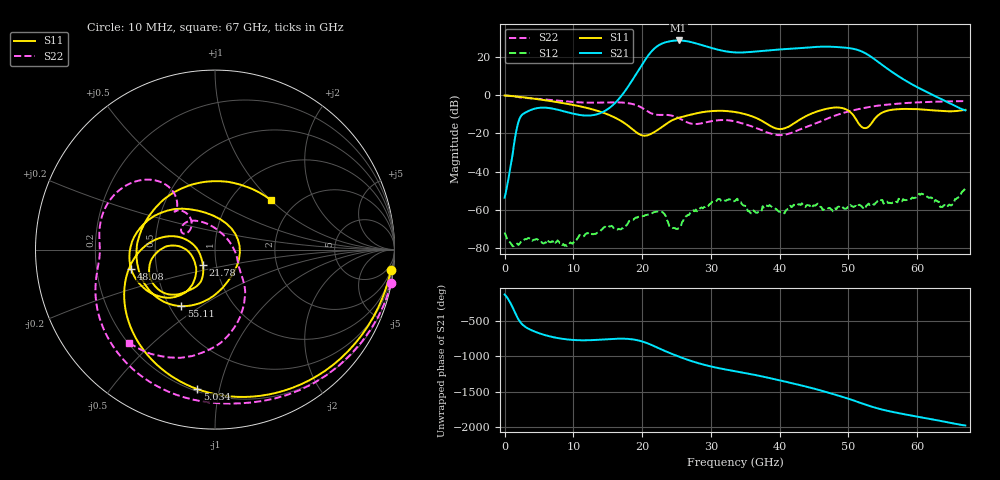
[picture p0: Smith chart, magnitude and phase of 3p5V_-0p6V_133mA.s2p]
! MARKI MICROWAVE INC.
! Date:  10/23/18
! Model Number:  AMM-6702CH
! Description:  2-port Small Signal S-parameter data for AMM-6702CH
! Frequency Range:  10 MHz to 67 GHz
! Port Configuration:  PORT 1: Input
!  PORT 2: Output
! Bias Condition: Vd = +3.5V, Vg = -0.6V
! AMM-6702CH s2p files are only valid for small signal conditions (below -5 dBm input power)
!S2P File: Measurements: Mag<S11> Ang<S11>, Mag<S21> Ang<S21>, Mag<S12> Ang<S12>, Mag<S22> Ang<S22>!row 1
# Hz S  dB  R 50
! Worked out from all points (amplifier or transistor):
!   401 points, 10 MHz to 67 GHz, reference 50 ohm
!   highest |S21| = 28.8 dB at 25.3 GHz (marker M1)
!   |S21| within 3 dB of that: 22.21 GHz to 29.21 GHz (7 GHz wide, 27.2 % of centre)
!   unconditionally stable (mu >= 1): start of sweep to end of sweep
!   at 11.06 GHz: K = 3267.83, MAG = -6.6 dB, |S12| = -73.4 dB
!   at 33.51 GHz: K = 18.14, MAG = 23.3 dB, |S12| = -55.3 dB
!   at 67 GHz: K = 135.82, MAG = -4.0 dB, |S12| = -48.5 dB
!   S11 on the Smith chart (normalised r, x): 10 MHz: 2, -17; 5.034 GHz: 0.21, -0.86; 21.78 GHz: 0.86, -0.15; 48.08 GHz: 0.36, -0.10; 55.11 GHz: 0.57, -0.42; 67 GHz: 1.51, +1.00
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1e7  -0.12 -6.8  -53.66 -133.8  -71.87 -151.1  -0.02 -10.8
5.03425e9  -2.12 -97.2  -6.54 41.8  -76.28 -73.0  -1.89 -126.5
1.123082e10  -5.97 -165.5  -10.44 -57.1  -73.72 -169.1  -3.74 -174.3
1.977205e10  -20.69 -174.2  14.87 -67.0  -63.28 137.7  -6.12 129.6
2.178175e10  -19.24 -128.1  24.52 -140.5  -61.17 116.3  -9.96 131.7
2.245165e10  -17.67 -120.0  26.32 -170.4  -60.80 100.4  -10.26 135.8
2.362398e10  -14.72 -114.0  28.00 139.7  -65.27 66.9  -10.25 135.3
2.529872e10  -11.78 -120.9  28.76 75.1  -69.55 112.0  -11.88 128.0
2.697348e10  -10.22 -127.4  28.02 17.0  -61.73 142.7  -14.69 135.5
2.915065e10  -8.61 -139.1  25.82 -44.9  -58.51 101.0  -14.25 152.9
3.3505e10  -8.74 -169.4  22.49 -131.6  -55.33 50.1  -13.66 129.2
3.718945e10  -12.94 174.3  23.21 160.1  -61.29 -10.3  -17.99 94.0
4.037148e10  -17.60 -149.5  24.12 91.4  -61.24 24.6  -20.82 32.8
4.238118e10  -13.98 -124.5  24.57 45.9  -57.64 86.7  -18.66 -9.2
4.472582e10  -9.42 -129.3  25.24 -10.3  -58.66 -32.4  -15.44 -37.1
4.656805e10  -7.28 -146.2  25.53 -59.5  -59.35 -58.6  -12.75 -47.4
4.807532e10  -6.37 -167.2  25.37 -102.0  -59.22 -118.6  -10.59 -55.4
5.058745e10  -9.90 135.1  24.47 -178.0  -58.21 179.3  -7.93 -69.7
5.242968e10  -17.18 7.9  22.11 119.7  -59.50 -48.9  -6.51 -79.7
5.510928e10  -8.72 -120.7  15.41 43.6  -56.75 -0.6  -5.06 -93.4
5.594665e10  -7.80 -134.6  13.23 25.1  -56.29 23.9  -4.76 -97.0
6.7e10  -7.61 41.4  -7.89 -174.8  -48.50 81.0  -3.00 -132.6
